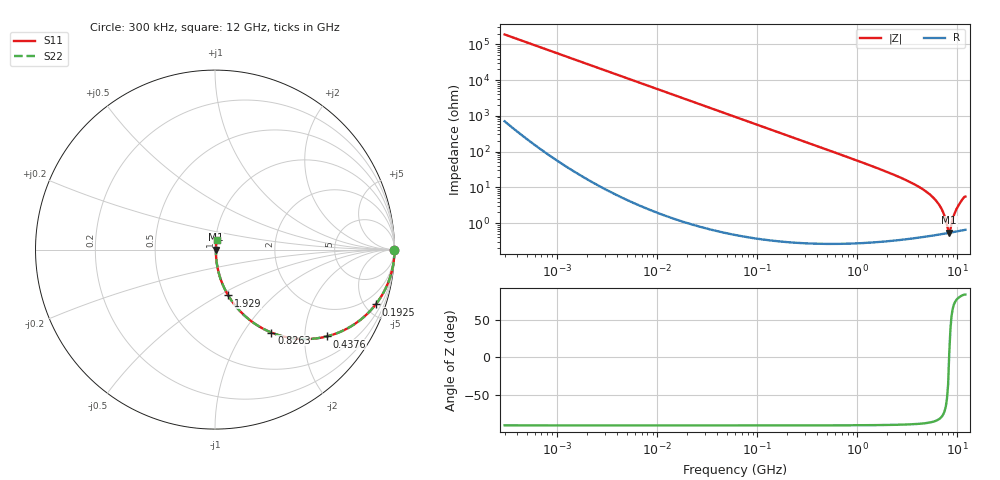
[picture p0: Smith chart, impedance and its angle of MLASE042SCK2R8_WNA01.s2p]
! MLASE042SCK2R8_WNA01  S-PARAMETER MODEL  ( General Type )
! Model Generated by TAIYO YUDEN Corporation (http://www.ty-top.com)
! Version 1.0
! TAIYO YUDEN Control No. 120810
! Copyright(c) 2012 TAIYO YUDEN CO.,LTD. All Rights Reserved.
! Product Description (link to TY-COMPAS)
! https://ds.yuden.co.jp/TYCOMPAS/or/detail?pn=MLASE042SCK2R8AWNA01&u=M
! Products Name : Multilayer Ceramic Capacitors
! Characteristics :
!  Capacitance : 2.8 pF , Rated Voltage : 16V , TCC : CK / C0K
!  Case Size : 0.4 x 0.2 / 0.016 x 0.008 [mm/inch] , Thickness : 0.2 / 0.008 [mm/inch]
!  (Conditions: Temperature = 25 degC , DC Bias Current/Voltage = 0A / 0V)
! External Node Assignments :
!  1  o---| |---o  2
! GND o---------o GND
! Frequency Range : 0.3MHz  -  12000MHz  [ 401 STEP ]
# MHz S RI R 50
! Freq[MHz].  S11 Real  S11 Imag  S21 Real  S21 Imag  S12 Real  S12 Imag  S22 Real  S22 Imag
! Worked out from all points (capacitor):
!   401 points, 300 kHz to 12 GHz, reference 50 ohm
!   read as one part in series: C = 2.82 pF near 316.3 kHz
!   lowest |Z| = 536 mohm at 8.282 GHz (marker M1)
!   series resonance near 8.255 GHz, so ESL is about 130 pH
!   S11 on the Smith chart (normalised r, x): 300 kHz: open; 192.5 MHz: 1.01, -5.86; 437.6 MHz: 1.01, -2.57; 826.3 MHz: 1.01, -1.35; 1.929 GHz: 1.01, -0.55; 12 GHz: 1.01, +0.11
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0.3  1 -0.000532  2.26e-06 0.000532  2.26e-06 0.000532  1 -0.000532
1.769972  1 -0.00314  1.19e-05 0.00314  1.19e-05 0.00314  1 -0.00314
10.44266  0.9997 -0.0185  0.000349 0.0185  0.000349 0.0185  0.9997 -0.0185
60  0.9888 -0.1051  0.0112 0.1051  0.0112 0.1051  0.9888 -0.1051
192.4766  0.8954 -0.3055  0.1046 0.3055  0.1046 0.3055  0.8954 -0.3055
353.9943  0.7165 -0.4499  0.2835 0.4499  0.2835 0.4499  0.7165 -0.4499
437.5599  0.6229 -0.4836  0.3771 0.4836  0.3771 0.4836  0.6229 -0.4836
826.3444  0.3144 -0.4623  0.6856 0.4623  0.6856 0.4623  0.3144 -0.4623
1262.535  0.1617 -0.3649  0.8383 0.3649  0.8383 0.3649  0.1617 -0.3649
1928.972  0.0735 -0.2555  0.9265 0.2555  0.9265 0.2555  0.0735 -0.2555
2088.533  0.0627 -0.2364  0.9373 0.2364  0.9373 0.2364  0.0627 -0.2364
3740.715  0.0178 -0.1175  0.9822 0.1175  0.9822 0.1175  0.0178 -0.1175
5420.343  0.00785 -0.0589  0.9921 0.0589  0.9921 0.0589  0.00785 -0.0589
6699.894  0.00564 -0.0289  0.9944 0.0289  0.9944 0.0289  0.00564 -0.0289
7254.098  0.0053 -0.018  0.9947 0.018  0.9947 0.018  0.0053 -0.018
7854.144  0.00523 -0.00726  0.9948 0.00726  0.9948 0.00726  0.00523 -0.00726
8281.503  0.00531 0.000534  0.9947 -0.000534  0.9947 -0.000534  0.00531 0.000534
8732.115  0.00551 0.00781  0.9945 -0.00781  0.9945 -0.00781  0.00551 0.00781
9207.246  0.00583 0.0153  0.9942 -0.0153  0.9942 -0.0153  0.00583 0.0153
9968.853  0.00653 0.0264  0.9935 -0.0264  0.9935 -0.0264  0.00653 0.0264
11083.22  0.00806 0.0433  0.9919 -0.0433  0.9919 -0.0433  0.00806 0.0433
12000  0.00935 0.0537  0.9906 -0.0537  0.9906 -0.0537  0.00935 0.0537
